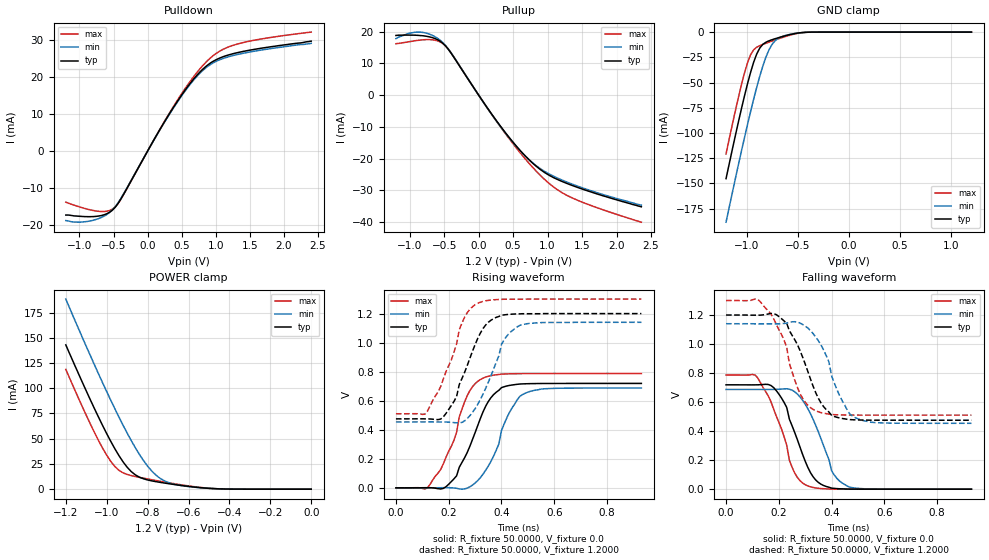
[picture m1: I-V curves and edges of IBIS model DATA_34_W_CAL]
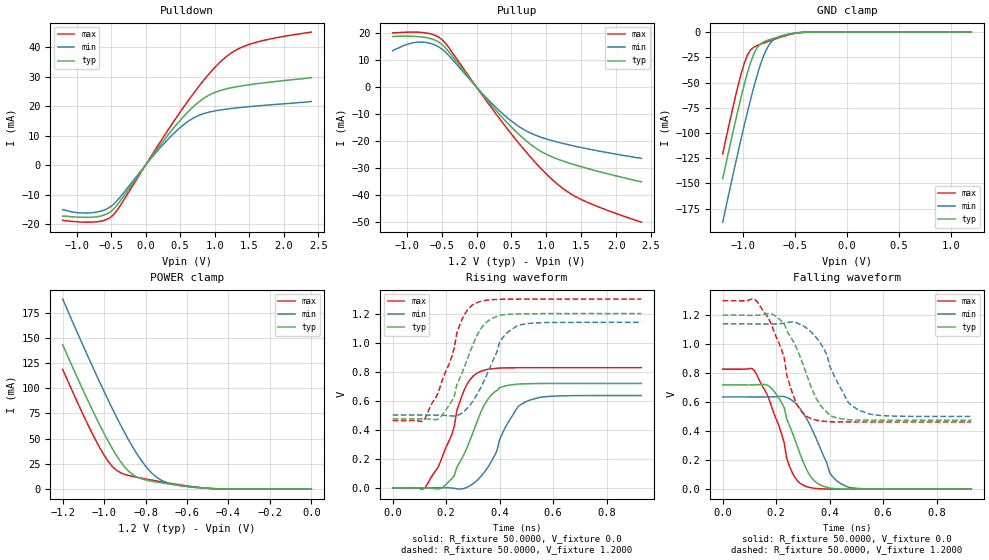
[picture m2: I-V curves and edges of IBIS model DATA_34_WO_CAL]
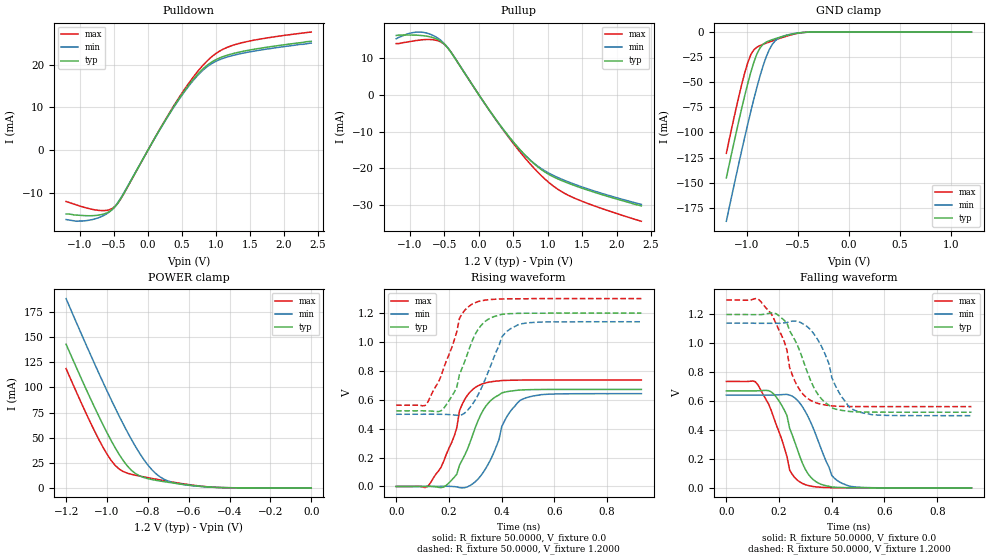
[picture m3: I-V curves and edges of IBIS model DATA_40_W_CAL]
| IBIS file uksl25616aa1.ibs created by s2ibis3 verion 3.2
| North Carolina State University, ERL, 2006
| This Model is valid for  Temperature Range -40C<=Tc<=125C
| Valid for LPDDR2-333/400/533/667/800/933/1066 operation
| Part Number   VDD2/VDDQ   Package   Architecture
| SCB4BL256160AFL19GA1  1.2 +0.1/-0.06V   FBGA-162   16Meg x 16
[IBIS Ver]   3.2
[File name]  usssl25616aa1.ibs
[File Rev]   1.1
[Date]   2022-02-17
[Source]   Simulation of a silicon level SPICE model
[Notes]   IBIS Characteristics for I/O Buffer
   IBIS Model Revision History:
Rev 1.0: 2018-01-17
   - IBIS model file initial creation
Rev 1.1: 2022-02-17
   - add pkg rlc
[disclaimer] The IBIS models are for modeling purpose only and are
   subject to change without any notice. UniIC is not
   responsible for any problems the models may cause.
[Copyright]  Copyright 2022 UniIC Semiconductors Corp. All rights reserved
|   Component SCB4BL256160AFL19GA1 (FBGA-162, x16)
[Component]   SCB4BL256160AFL19GA1
[Manufacturer]  UniIC Semiconductors Corp.
[Package]
|Variable   typ   min   max
R_pkg   0.556   0.378   0.679
L_pkg   1.908nH   1.302nH   2.216nH
C_pkg   0.582pF   0.372pF   0.754pF
[Pin]   signal_name   model_name   R_pin   L_pin   C_pin
E5	VDD2		POWER		NA		NA		NA
E6	VDD1		POWER		NA		NA		NA
F1	VDD1		POWER		NA		NA		NA
F2	VSS		GND		NA		NA		NA
F5	VSS		GND		NA		NA		NA
F6	VSSQ		GND		NA		NA		NA
F7	VDDQ		POWER		NA		NA		NA
F9	VSSQ		GND		NA		NA		NA
F10	VDDQ		POWER		NA		NA		NA
G1	VSS		GND		NA		NA		NA
G2	VDD2		POWER		NA		NA		NA
G3	ZQ0		NC
G5	VDDQ		POWER		NA		NA		NA
G10	VSSQ		GND		NA		NA		NA
H1	VSS		GND		NA		NA		NA
H2	CA9		CLKCA_RCV	0.474		1.978nH		0.453pF
H3	CA8		CLKCA_RCV	0.460		1.859nH		0.433pF
H8	DQ15		DQ		0.640		2.088nH		0.676pF
H9	VDDQ		POWER		NA		NA		NA
H10	VSSQ		GND		NA		NA		NA
J1	VDDCA		POWER		NA		NA		NA
J2	CA6		CLKCA_RCV	0.471		1.976nH		0.469pF
J3	CA7		CLKCA_RCV	0.458		1.961nH		0.412pF
J5	VSSQ		GND		NA		NA		NA
J6	DQ11		DQ		0.620		1.893nH		0.688pF
J7	DQ13		DQ		0.643		2.053nH		0.667pF
J8	DQ14		DQ		0.633		2.077nH		0.656pF
J9	DQ12		DQ		0.592		1.879nH		0.569pF
J10	VDDQ		POWER		NA		NA		NA
K1	VDD2		POWER		NA		NA		NA
K2	CA5		CLKCA_RCV	0.464		1.759nH		0.443pF
K3	VrefCA		NC
K5	DQS1_c		DQ		0.679		2.216nH		0.754pF
K6	DQS1_t		DQ		0.674		2.149nH		0.750pF
K7	DQ10		DQ		0.597		1.926nH		0.614pF
K8	DQ9		DQ		0.587		1.830nH		0.662pF
K9	DQ8		DQ		0.579		1.883nH		0.630pF
K10	VSSQ		GND		NA		NA		NA
L1	VDDCA		POWER		NA		NA		NA
L2	VSS		GND		NA		NA		NA
L3	CK_c		CLKCA_RCV	0.378		1.454nH		0.372pF
L5	DM1		DQ		0.651		1.935nH		0.742pF
L6	VDDQ		POWER		NA		NA		NA
M1	VSS		GND		NA		NA		NA
M3	CK_t		CLKCA_RCV	0.389		1.302nH		0.400pF
M5	VSSQ		GND		NA		NA		NA
M6	VDDQ		POWER		NA		NA		NA
M7	VDD2		POWER		NA		NA		NA
M8	VSS		GND		NA		NA		NA
M9	VrefDQ		NC
N1	CKE		CLKCA_RCV	0.446		1.614nH		0.442pF
N5	DM0		DQ		0.641		1.892nH		0.746pF
N6	VDDQ		POWER		NA		NA		NA
P1	CS_n		CLKCA_RCV	0.447		1.842nH		0.456pF
P5	DQS0_c		DQ		0.648		2.065nH		0.741pF
P6	DQS0_t		DQ		0.647		2.022nH		0.742pF
P7	DQ5		DQ		0.600		2.057nH		0.612pF
P8	DQ6		DQ		0.585		1.896nH		0.623pF
P9	DQ7		DQ		0.578		1.887nH		0.582pF
P10	VSSQ		GND		NA		NA		NA
R1	CA4		CLKCA_RCV	0.464		1.944nH		0.462pF
R2	CA3		CLKCA_RCV	0.448		2.047nH		0.405pF
R3	CA2		CLKCA_RCV	0.448		1.881nH		0.471pF
R5	VSSQ		GND		NA		NA		NA
R6	DQ4		DQ		0.623		1.911nH		0.703pF
R7	DQ2		DQ		0.641		1.973nH		0.688pF
R8	DQ1		DQ		0.632		2.051nH		0.649pF
R9	DQ3		DQ		0.598		1.884nH		0.594pF
R10	VDDQ		POWER		NA		NA		NA
T1	VSS		GND		NA		NA		NA
T2	VDDCA		POWER		NA		NA		NA
T3	CA1		CLKCA_RCV	0.470		1.857nH		0.486pF
T8	DQ0		DQ		0.629		2.028nH		0.661pF
T9	VDDQ		POWER		NA		NA		NA
T10	VSSQ		GND		NA		NA		NA
U1	VSS		GND		NA		NA		NA
U2	VDD2		POWER		NA		NA		NA
U3	CA0		CLKCA_RCV	0.487		1.606nH		0.509pF
U5	VDDQ		POWER		NA		NA		NA
U10	VSSQ		GND		NA		NA		NA
V1	VDD1		POWER		NA		NA		NA
V2	VSS		GND		NA		NA		NA
V5	VSS		GND		NA		NA		NA
V6	VSSQ		GND		NA		NA		NA
V7	VDDQ		POWER		NA		NA		NA
V9	VSSQ		GND		NA		NA		NA
V10	VDDQ		POWER		NA		NA		NA
W5	VDD2		POWER		NA		NA		NA
W6	VDD1		POWER		NA		NA		NA
|*****************************  Diff Pin  *************************************
[Diff Pin]  inv_pin  vdiff   tdelay_typ  tdelay_min  tdelay_max
M3   L3   0.44000V   NA   NA   NA
P6   P5   0.44000V   NA   NA   NA
K6   K5   0.44000V   NA   NA   NA
|*****************************  Model Selector ********************************
[Model Selector]   DQ
DATA_34_W_CAL   RZQ/7 Output Driver, With ZQ Cal
DATA_40_W_CAL   RZQ/6 Output Driver, With ZQ Cal
DATA_48_W_CAL   RZQ/5 Output Driver, With ZQ Cal
DATA_60_W_CAL   RZQ/4 Output Driver, With ZQ Cal
DATA_80_W_CAL   RZQ/3 Output Driver, With ZQ Cal
DATA_120_W_CAL   RZQ/2 Output Driver, With ZQ Cal
DATA_34_WO_CAL   RZQ/7 Output Driver, Without ZQ Cal
DATA_40_WO_CAL   RZQ/6 Output Driver, Without ZQ Cal
DATA_48_WO_CAL   RZQ/5 Output Driver, Without ZQ Cal
DATA_60_WO_CAL   RZQ/4 Output Driver, Without ZQ Cal
DATA_80_WO_CAL   RZQ/3 Output Driver, Without ZQ Cal
DATA_120_WO_CAL   RZQ/2 Output Driver, Without ZQ Cal
DATA_RCV   Data/Data Strobe/Data Mask Receiver
| Models and submodels in the file (14): DATA_34_W_CAL (I/O), DATA_34_WO_CAL (I/O), DATA_40_W_CAL (I/O), DATA_40_WO_CAL (I/O), DATA_48_W_CAL (I/O), DATA_48_WO_CAL (I/O), DATA_60_W_CAL (I/O), DATA_60_WO_CAL (I/O), DATA_80_W_CAL (I/O), DATA_80_WO_CAL (I/O), DATA_120_W_CAL (I/O), DATA_120_WO_CAL (I/O), DATA_RCV (Input), CLKCA_RCV (Input)
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|   Model DATA_34_W_CAL
[Model]  DATA_34_W_CAL
Model_type I/O
Polarity   Non-Inverting
Enable   Active-High
Vinl =   0.3800V
Vinh =   0.8200V
Vmeas =  0.6000V
Cref =   5.0000pF
Rref =   50.0000
Vref =   0.6000V
C_comp   1.7430pF   1.7110pF   1.7640pF
[Temperature Range]   25.0000   0.1250k   -40.0000
[Voltage Range]   1.2000V   1.1400V   1.3000V
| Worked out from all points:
|   slope of the pulldown table from 0 to 0.18 V, typ, clamps not added: 31 ohm
|   slope of the pullup table from 0 to 0.18 V, typ, clamps not added: 31.6 ohm
|   GND clamp passes 1 mA (typ) near -0.50 V on its own axis
|   POWER clamp passes 1 mA (typ) near -0.51 V on its own axis
|   rising waveform, R_fixture 50.0000, V_fixture 0.0: 20-80 % time 103ps typ, 94.1ps min, 91.3ps max; typ from 0 V to 0.719 V
|   rising waveform, R_fixture 50.0000, V_fixture 1.2000: 20-80 % time 89.8ps typ, 90ps min, 90.2ps max; typ from 0.475 V to 1.2 V
|   falling waveform, R_fixture 50.0000, V_fixture 0.0: 20-80 % time 85.3ps typ, 87.3ps min, 85.5ps max; typ from 0.719 V to 0 V
|   falling waveform, R_fixture 50.0000, V_fixture 1.2000: 20-80 % time 99.7ps typ, 89.3ps min, 89.4ps max; typ from 1.2 V to 0.475 V
[Pulldown]
|Voltage   I(typ)   I(min)   I(max)
-1.2V     -17.3mA    -18.8mA    -13.8mA
-1V       -17.63mA   -19.23mA   -15.09mA
-760mV    -17.66mA   -18.52mA   -16.19mA
-600mV    -16.96mA   -17.17mA   -16.27mA
-480mV    -15.3mA    -15.16mA   -15.18mA
-360mV    -11.96mA   -11.8mA    -12.01mA
400mV     12.41mA    12.24mA    12.65mA
680mV     19.58mA    19.29mA    20.22mA
880mV     23.24mA    22.86mA    24.47mA
1.08V     25.31mA    24.84mA    27.24mA
1.32V     26.61mA    26.11mA    28.94mA
2.4V      29.7mA     29.1mA     32.16mA
[Pullup]
|Voltage   I(typ)   I(min)   I(max)
-1.2V     18.8mA     17.8mA     16.2mA
-1.04V    18.92mA    19.3mA     16.72mA
-840mV    18.77mA    19.84mA    17.37mA
-680mV    18.18mA    18.92mA    17.46mA
-520mV    16.35mA    16.56mA    16.27mA
-400mV    13.24mA    13.33mA    13.31mA
320mV     -9.896mA   -10.02mA   -10.1mA
560mV     -16.42mA   -16.51mA   -17.03mA
800mV     -21.78mA   -21.65mA   -23.17mA
1.04V     -25.48mA   -25.07mA   -28.17mA
1.28V     -27.85mA   -27.42mA   -31.61mA
2.36V     -35.2mA    -34.7mA    -40.07mA
[GND_clamp]
|Voltage   I(typ)   I(min)   I(max)
-1.2V     -145.3mA   -188.5mA   -120.8mA
-1.05V    -76.2mA    -118.2mA   -52.43mA
-990mV    -51.2mA    -91.62mA   -30.39mA
-960mV    -39.9mA    -78.82mA   -22.48mA
-900mV    -21.67mA   -54.7mA    -15mA
-870mV    -15.78mA   -43.66mA   -13.45mA
-810mV    -10.04mA   -24.79mA   -11.07mA
-780mV    -8.658mA   -17.59mA   -9.958mA
-720mV    -6.57mA    -8.545mA   -7.793mA
-630mV    -3.906mA   -3.64mA    -4.741mA
-420mV    -215.4uA   -240.5uA   -235uA
1.2V      1.597nA    22.84nA    1.463nA
[POWER_clamp]
|Voltage   I(typ)   I(min)   I(max)
-1.2V     143mA      188.4mA    118.7mA
-1.1V     97.38mA    141.5mA    73.24mA
-1.04V    71.38mA    114.3mA    48.22mA
-1V       55.04mA    96.69mA    33.64mA
-960mV    40mA       79.65mA    22.42mA
-900mV    21.75mA    55.6mA     14.58mA
-860mV    14.17mA    41.05mA    12.52mA
-800mV    9.133mA    22.79mA    10.12mA
-740mV    6.786mA    10.88mA    7.886mA
-660mV    4.332mA    4.436mA    5.101mA
-520mV    1.103mA    1.063mA    1.274mA
0V        1.597nA    6.003nA    2.16nA
[Ramp]
| variable   typ   min   max
dV/dt_r  0.4314/96.1802p   0.4123/96.8370p   0.4720/94.2430p
dV/dt_f  0.4350/92.7485p   0.4117/92.3765p   0.4739/92.4509p
R_load = 50.0000
[Rising Waveform]
R_fixture= 50.0000
V_fixture= 0.0
V_fixture_min= 0.0
V_fixture_max= 0.0
|time   V(typ)   V(min)   V(max)
0s        0V         0V         0V
120ps     1.003mV    148uV      1.23mV
190ps     8.093mV    1.237mV    212mV
230ps     83.25mV    -2.991mV   383.2mV
270ps     242.6mV    -2.242mV   634.2mV
330ps     522.8mV    94.41mV    755.5mV
380ps     658.4mV    259mV      778.6mV
400ps     690mV      394.3mV    783.1mV
480ps     715.9mV    642.4mV    786.4mV
930ps     719mV      687.2mV    786.7mV
[Rising Waveform]
R_fixture= 50.0000
V_fixture= 1.2000
V_fixture_min= 1.1400
V_fixture_max= 1.3000
|time   V(typ)   V(min)   V(max)
0s        475mV      453.9mV    510.1mV
110ps     475mV      454.1mV    507.6mV
180ps     489.3mV    453.5mV    751.9mV
230ps     629.5mV    447.7mV    991.9mV
260ps     794.2mV    460.8mV    1.174V
310ps     1.029V     574.7mV    1.271V
350ps     1.14V      726.5mV    1.291V
400ps     1.189V     987.9mV    1.298V
470ps     1.198V     1.119V     1.299V
930ps     1.2V       1.14V      1.3V
[Falling Waveform]
R_fixture= 50.0000
V_fixture= 0.0
V_fixture_min= 0.0
V_fixture_max= 0.0
|time   V(typ)   V(min)   V(max)
0s        719mV      687.2mV    786.7mV
110ps     718.8mV    687mV      786.5mV
180ps     700.3mV    687.2mV    553.5mV
230ps     562.6mV    691.8mV    302.3mV
250ps     437.6mV    682.4mV    151.9mV
310ps     150mV      554.3mV    22.24mV
350ps     46.23mV    393.3mV    5.968mV
400ps     7.106mV    126.7mV    822.2uV
460ps     926.8uV    20.72mV    95.79uV
930ps     0V         0V         0V
[Falling Waveform]
R_fixture= 50.0000
V_fixture= 1.2000
V_fixture_min= 1.1400
V_fixture_max= 1.3000
|time   V(typ)   V(min)   V(max)
0s        1.2V       1.14V      1.3V
120ps     1.199V     1.139V     1.308V
210ps     1.175V     1.141V     1.066V
280ps     956.7mV    1.145V     660.1mV
340ps     664mV      1.048V     540.2mV
390ps     531.3mV    875.3mV    517.7mV
400ps     508.8mV    780.4mV    514.4mV
460ps     481.3mV    542.9mV    510.8mV
490ps     477.5mV    492.5mV    510.4mV
930ps     475mV      453.9mV    510.1mV
|   Model DATA_34_WO_CAL
[Model]  DATA_34_WO_CAL
Model_type I/O
Polarity   Non-Inverting
Enable   Active-High
Vinl =   0.3800V
Vinh =   0.8200V
Vmeas =  0.6000V
Cref =   5.0000pF
Rref =   50.0000
Vref =   0.6000V
C_comp   1.7430pF   1.7110pF   1.7640pF
[Temperature Range]   25.0000   0.1250k   -40.0000
[Voltage Range]   1.2000V   1.1400V   1.3000V
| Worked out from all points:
|   slope of the pulldown table from 0 to 0.18 V, typ, clamps not added: 31 ohm
|   slope of the pullup table from 0 to 0.18 V, typ, clamps not added: 31.6 ohm
|   GND clamp passes 1 mA (typ) near -0.50 V on its own axis
|   POWER clamp passes 1 mA (typ) near -0.51 V on its own axis
|   rising waveform, R_fixture 50.0000, V_fixture 0.0: 20-80 % time 103ps typ, 101ps min, 89.8ps max; typ from 0 V to 0.719 V
|   rising waveform, R_fixture 50.0000, V_fixture 1.2000: 20-80 % time 89.8ps typ, 92.2ps min, 89.9ps max; typ from 0.475 V to 1.2 V
|   falling waveform, R_fixture 50.0000, V_fixture 0.0: 20-80 % time 85.3ps typ, 91.3ps min, 84.8ps max; typ from 0.719 V to 0 V
|   falling waveform, R_fixture 50.0000, V_fixture 1.2000: 20-80 % time 99.7ps typ, 97.1ps min, 84.6ps max; typ from 1.2 V to 0.475 V
[Pulldown]
|Voltage   I(typ)   I(min)   I(max)
-1.2V     -17.3mA    -15.1mA    -18.7mA
-1V       -17.63mA   -16.13mA   -19.23mA
-760mV    -17.66mA   -16.12mA   -19.34mA
-600mV    -16.96mA   -15.26mA   -18.76mA
-480mV    -15.3mA    -13.63mA   -17.17mA
-360mV    -11.96mA   -10.64mA   -13.5mA
200mV     6.437mA    5.606mA    7.408mA
520mV     15.7mA     13.13mA    18.66mA
840mV     22.64mA    17.47mA    28.77mA
1.2V      26.05mA    19.1mA     37.38mA
1.6V      27.6mA     20.06mA    41.68mA
2.4V      29.7mA     21.6mA     45.16mA
[Pullup]
|Voltage   I(typ)   I(min)   I(max)
-1.2V     18.8mA     13.5mA     20.2mA
-840mV    18.77mA    16.72mA    20.41mA
-680mV    18.18mA    16.36mA    19.94mA
-520mV    16.35mA    14.59mA    18.19mA
-400mV    13.24mA    11.8mA     14.79mA
80mV      -2.576mA   -2.297mA   -2.91mA
360mV     -11.05mA   -9.571mA   -12.76mA
600mV     -17.41mA   -14.52mA   -20.69mA
840mV     -22.52mA   -17.84mA   -27.96mA
1.12V     -26.37mA   -20.16mA   -35.21mA
1.4V      -28.83mA   -21.92mA   -40.43mA
2.36V     -35.2mA    -26.5mA    -50.22mA
[GND_clamp]
|Voltage   I(typ)   I(min)   I(max)
-1.2V     -145.3mA   -188.5mA   -120.8mA
-1.05V    -76.2mA    -118.2mA   -52.43mA
-990mV    -51.2mA    -91.62mA   -30.39mA
-960mV    -39.9mA    -78.82mA   -22.48mA
-900mV    -21.67mA   -54.7mA    -15mA
-870mV    -15.78mA   -43.66mA   -13.45mA
-810mV    -10.04mA   -24.79mA   -11.07mA
-780mV    -8.658mA   -17.59mA   -9.958mA
-720mV    -6.57mA    -8.545mA   -7.793mA
-630mV    -3.906mA   -3.64mA    -4.741mA
-420mV    -215.4uA   -240.5uA   -235uA
1.2V      1.597nA    22.84nA    1.463nA
[POWER_clamp]
|Voltage   I(typ)   I(min)   I(max)
-1.2V     143mA      188.4mA    118.7mA
-1.1V     97.38mA    141.5mA    73.24mA
-1.04V    71.38mA    114.3mA    48.22mA
-1V       55.04mA    96.69mA    33.64mA
-960mV    40mA       79.65mA    22.42mA
-900mV    21.75mA    55.6mA     14.58mA
-860mV    14.17mA    41.05mA    12.52mA
-800mV    9.133mA    22.79mA    10.12mA
-740mV    6.786mA    10.88mA    7.886mA
-660mV    4.332mA    4.436mA    5.101mA
-520mV    1.103mA    1.063mA    1.274mA
0V        1.597nA    6.003nA    2.16nA
[Ramp]
| variable   typ   min   max
dV/dt_r  0.4314/96.1802p   0.3815/0.1044n   0.4965/92.7944p
dV/dt_f  0.4350/92.7485p   0.3830/0.1043n   0.5020/88.0000p
R_load = 50.0000
[Rising Waveform]
R_fixture= 50.0000
V_fixture= 0.0
V_fixture_min= 0.0
V_fixture_max= 0.0
|time   V(typ)   V(min)   V(max)
0s        0V         0V         0V
120ps     1.003mV    147uV      141.1uV
180ps     -3.556mV   1.093mV    185.9mV
230ps     83.25mV    -2.659mV   420.7mV
240ps     141.6mV    -6.697mV   533.8mV
270ps     242.6mV    -1.943mV   684.9mV
320ps     477.7mV    59.6mV     794.5mV
400ps     690mV      334.3mV    825.2mV
490ps     716.6mV    585.6mV    827.4mV
930ps     719mV      635.9mV    827.5mV
[Rising Waveform]
R_fixture= 50.0000
V_fixture= 1.2000
V_fixture_min= 1.1400
V_fixture_max= 1.3000
|time   V(typ)   V(min)   V(max)
0s        475mV      501.6mV    463.3mV
110ps     475mV      501.9mV    457.1mV
180ps     489.3mV    500.3mV    709.4mV
230ps     629.5mV    494.5mV    962.8mV
260ps     794.2mV    516.1mV    1.163V
310ps     1.029V     626.6mV    1.271V
350ps     1.14V      771mV      1.292V
400ps     1.189V     1.004V     1.298V
470ps     1.198V     1.119V     1.299V
930ps     1.2V       1.14V      1.3V
[Falling Waveform]
R_fixture= 50.0000
V_fixture= 0.0
V_fixture_min= 0.0
V_fixture_max= 0.0
|time   V(typ)   V(min)   V(max)
0s        719mV      635.9mV    827.5mV
120ps     719.1mV    635.7mV    814.7mV
170ps     714.5mV    636mV      637.9mV
210ps     628.4mV    638.9mV    438.2mV
250ps     437.6mV    623.6mV    157.9mV
300ps     192.5mV    528mV      28.39mV
340ps     62.78mV    389.2mV    6.858mV
400ps     7.106mV    113.2mV    563uV
460ps     926.8uV    20.53mV    55.08uV
930ps     0V         0V         0V
[Falling Waveform]
R_fixture= 50.0000
V_fixture= 1.2000
V_fixture_min= 1.1400
V_fixture_max= 1.3000
|time   V(typ)   V(min)   V(max)
0s        1.2V       1.14V      1.3V
130ps     1.199V     1.139V     1.29V
230ps     1.142V     1.144V     905.3mV
240ps     1.092V     1.149V     783mV
270ps     997.7mV    1.15V      616.5mV
320ps     758.6mV    1.102V     495.9mV
370ps     567.9mV    993.6mV    469.8mV
400ps     508.8mV    849.7mV    465.1mV
500ps     477mV      555.1mV    463.3mV
930ps     475mV      501.6mV    463.3mV
|   Model DATA_40_W_CAL
[Model]  DATA_40_W_CAL
Model_type I/O
Polarity   Non-Inverting
Enable   Active-High
Vinl =   0.3800V
Vinh =   0.8200V
Vmeas =  0.6000V
Cref =   5.0000pF
Rref =   50.0000
Vref =   0.6000V
C_comp   1.7430pF   1.7110pF   1.7640pF
[Temperature Range]   25.0000   0.1250k   -40.0000
[Voltage Range]   1.2000V   1.1400V   1.3000V
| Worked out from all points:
|   slope of the pulldown table from 0 to 0.18 V, typ, clamps not added: 36.2 ohm
|   slope of the pullup table from 0 to 0.18 V, typ, clamps not added: 36.7 ohm
|   GND clamp passes 1 mA (typ) near -0.50 V on its own axis
|   POWER clamp passes 1 mA (typ) near -0.51 V on its own axis
|   rising waveform, R_fixture 50.0000, V_fixture 0.0: 20-80 % time 95.4ps typ, 89.9ps min, 82.6ps max; typ from 0 V to 0.672 V
|   rising waveform, R_fixture 50.0000, V_fixture 1.2000: 20-80 % time 81.5ps typ, 87.6ps min, 82.8ps max; typ from 0.523 V to 1.2 V
|   falling waveform, R_fixture 50.0000, V_fixture 0.0: 20-80 % time 77.9ps typ, 88.3ps min, 80.1ps max; typ from 0.672 V to 0 V
|   falling waveform, R_fixture 50.0000, V_fixture 1.2000: 20-80 % time 96.1ps typ, 87.4ps min, 83.4ps max; typ from 1.2 V to 0.523 V
[Pulldown]
|Voltage   I(typ)   I(min)   I(max)
-1.2V     -14.8mA    -16.1mA    -11.9mA
-1.04V    -15.06mA   -16.5mA    -12.74mA
-800mV    -15.19mA   -16.05mA   -13.77mA
-600mV    -14.54mA   -14.72mA   -13.95mA
-480mV    -13.11mA   -13mA      -13.01mA
-360mV    -10.25mA   -10.12mA   -10.29mA
400mV     10.64mA    10.49mA    10.85mA
680mV     16.78mA    16.53mA    17.33mA
880mV     19.92mA    19.59mA    20.97mA
1.08V     21.7mA     21.29mA    23.35mA
1.32V     22.81mA    22.38mA    24.81mA
2.4V      25.4mA     25mA       27.56mA
[Pullup]
|Voltage   I(typ)   I(min)   I(max)
-1.2V     16.1mA     15.2mA     13.9mA
-1V       16.22mA    16.71mA    14.45mA
-840mV    16.09mA    17.01mA    14.89mA
-680mV    15.59mA    16.24mA    14.97mA
-520mV    14.05mA    14.23mA    13.98mA
-400mV    11.39mA    11.47mA    11.45mA
320mV     -8.514mA   -8.621mA   -8.69mA
560mV     -14.12mA   -14.2mA    -14.65mA
800mV     -18.71mA   -18.6mA    -19.92mA
1.04V     -21.88mA   -21.52mA   -24.2mA
1.28V     -23.9mA    -23.53mA   -27.13mA
2.36V     -30.2mA    -29.8mA    -34.37mA
[GND_clamp]
|Voltage   I(typ)   I(min)   I(max)
-1.2V     -145.3mA   -188.5mA   -120.8mA
-1.05V    -76.2mA    -118.2mA   -52.43mA
-990mV    -51.2mA    -91.62mA   -30.39mA
-960mV    -39.9mA    -78.82mA   -22.48mA
-900mV    -21.67mA   -54.7mA    -15mA
-870mV    -15.78mA   -43.66mA   -13.45mA
-810mV    -10.04mA   -24.79mA   -11.07mA
-780mV    -8.658mA   -17.59mA   -9.958mA
-720mV    -6.57mA    -8.545mA   -7.793mA
-630mV    -3.906mA   -3.64mA    -4.741mA
-420mV    -215.4uA   -240.5uA   -235uA
1.2V      1.597nA    22.84nA    1.463nA
[POWER_clamp]
|Voltage   I(typ)   I(min)   I(max)
-1.2V     143mA      188.4mA    118.7mA
-1.1V     97.38mA    141.5mA    73.24mA
-1.04V    71.38mA    114.3mA    48.22mA
-1V       55.04mA    96.69mA    33.64mA
-960mV    40mA       79.65mA    22.42mA
-900mV    21.75mA    55.6mA     14.58mA
-860mV    14.17mA    41.05mA    12.52mA
-800mV    9.133mA    22.79mA    10.12mA
-740mV    6.786mA    10.88mA    7.886mA
-660mV    4.332mA    4.436mA    5.101mA
-520mV    1.103mA    1.063mA    1.274mA
0V        1.597nA    6.003nA    2.16nA
[Ramp]
| variable   typ   min   max
dV/dt_r  0.4030/90.3786p   0.3853/92.8644p   0.4419/86.1430p
dV/dt_f  0.4060/89.3830p   0.3842/90.6269p   0.4427/86.8818p
R_load = 50.0000
[Rising Waveform]
R_fixture= 50.0000
V_fixture= 0.0
V_fixture_min= 0.0
V_fixture_max= 0.0
|time   V(typ)   V(min)   V(max)
0s        0V         0V         0V
120ps     1.042mV    148.4uV    1.036mV
190ps     7.806mV    1.304mV    221.7mV
220ps     63.13mV    -1.024mV   348.2mV
250ps     182mV      -9.492mV   567.3mV
320ps     494mV      71.85mV    704.7mV
370ps     611.7mV    233.3mV    727mV
410ps     651.9mV    450.5mV    733.7mV
470ps     667.5mV    595.9mV    736mV
930ps     671.6mV    642.2mV    736.5mV
[Rising Waveform]
R_fixture= 50.0000
V_fixture= 1.2000
V_fixture_min= 1.1400
V_fixture_max= 1.3000
|time   V(typ)   V(min)   V(max)
0s        523.4mV    499.6mV    562.2mV
110ps     523.3mV    499.9mV    560.7mV
180ps     539.9mV    498.9mV    817.8mV
230ps     688.5mV    492.6mV    1.072V
240ps     775.7mV    492.4mV    1.163V
300ps     1.054V     599.2mV    1.272V
340ps     1.146V     751.7mV    1.29V
400ps     1.191V     1.033V     1.298V
460ps     1.198V     1.117V     1.299V
930ps     1.2V       1.14V      1.3V
[Falling Waveform]
R_fixture= 50.0000
V_fixture= 0.0
V_fixture_min= 0.0
V_fixture_max= 0.0
|time   V(typ)   V(min)   V(max)
0s        671.6mV    642.2mV    736.5mV
110ps     671.5mV    642mV      734.5mV
180ps     649.1mV    642.4mV    484.9mV
230ps     500.3mV    646.9mV    216.4mV
240ps     413.2mV    642.3mV    124.1mV
290ps     165mV      557.8mV    29.18mV
330ps     56.08mV    411.7mV    9.051mV
400ps     5.96mV     85.76mV    863.2uV
440ps     1.927mV    30.36mV    265.5uV
930ps     0V         0V         0V
[Falling Waveform]
R_fixture= 50.0000
V_fixture= 1.2000
V_fixture_min= 1.1400
V_fixture_max= 1.3000
|time   V(typ)   V(min)   V(max)
0s        1.2V       1.14V      1.3V
120ps     1.199V     1.139V     1.308V
200ps     1.191V     1.139V     1.091V
230ps     1.141V     1.144V     953.9mV
260ps     1.023V     1.155V     738.7mV
330ps     702.2mV    1.071V     596mV
370ps     598.6mV    945.2mV    575mV
420ps     542.6mV    684.4mV    565.1mV
480ps     527.2mV    542.9mV    562.7mV
930ps     523.4mV    499.6mV    562.2mV
